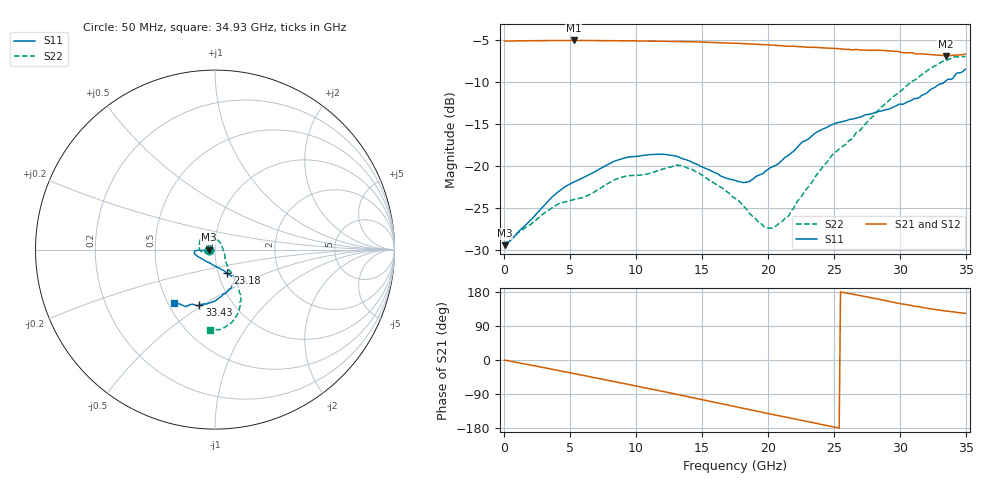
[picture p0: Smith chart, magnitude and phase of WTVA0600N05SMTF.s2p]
! 50 ohm 2-Port S-parameters measured by Modelithics Inc support@modelithics.com  Tampa, FL USA 813-866-6335 (February 2024)
! Smiths Interconnect,  6dB P/N: WTVA0600N05SMTF, Temperature: 50 C
! Board: 10 mil Rogers 4350B, Mounting Pad Dimensions: Length: 15 mils, Width: 25 mils, Gap: 40 mils.
# Hz S RI R 50
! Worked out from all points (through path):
!   352 points, 50 MHz to 34.93 GHz, reference 50 ohm
!   highest |S21| = -5.06 dB at 5.274 GHz (marker M1); lowest = -6.9 dB at 33.43 GHz (marker M2)
!   group delay of S21, straight-line fit = 19.5 ps
!   lowest |S11| = -29.5 dB at 50 MHz (marker M3), VSWR 1.07, Z = 46.7 - j0.0123 ohm
!   |S11| at or under -10 dB: start of sweep to 33.34 GHz
!   |S22| runs from -29.5 to -7.0 dB; largest |S21 - S12| = 0.006
!   S11 on the Smith chart (normalised r, x): 50 MHz: 0.93, -0.00; 23.18 GHz: 1.11, -0.30; 33.43 GHz: 0.70, -0.48; 34.93 GHz: 0.54, -0.37
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5e7  -0.0337 -0.000131  0.5542 -0.00272  0.5539 -0.00284  -0.0333 -0.00208
1.0955e9  -0.0404 -0.00414  0.5509 -0.0696  0.5506 -0.0696  -0.0395 -0.00774
3.4835e9  -0.0633 -0.00499  0.5121 -0.2202  0.5115 -0.2205  -0.0529 -0.0158
5.2745e9  -0.0801 -0.00379  0.4535 -0.3256  0.4532 -0.325  -0.0609 -0.0164
5.8715e9  -0.0842 -0.00353  0.4288 -0.3571  0.4284 -0.3568  -0.0626 -0.0154
8.757e9  -0.1092 -0.00599  0.2792 -0.4805  0.2783 -0.4804  -0.0849 -0.00182
1.1742e10  -0.1158 -0.0196  0.087 -0.5452  0.0859 -0.5448  -0.0864 0.0382
1.36325e10  -0.1057 -0.0303  -0.0444 -0.5486  -0.0452 -0.548  -0.0726 0.0679
1.48265e10  -0.0916 -0.0405  -0.1267 -0.5321  -0.1276 -0.5312  -0.0513 0.074
1.7513e10  -0.0485 -0.0661  -0.293 -0.4513  -0.293 -0.4506  -0.00151 0.064
1.8508e10  -0.0244 -0.0767  -0.3448 -0.406  -0.3449 -0.4053  0.0181 0.05
1.9702e10  0.00103 -0.0914  -0.3981 -0.3455  -0.3979 -0.3448  0.0361 0.0242
2.0299e10  0.0113 -0.0979  -0.4213 -0.3118  -0.4209 -0.3115  0.0408 0.0122
2.1493e10  0.0348 -0.1097  -0.4547 -0.2439  -0.4546 -0.2429  0.0483 -0.0128
2.31845e10  0.0687 -0.131  -0.4884 -0.1421  -0.4878 -0.1422  0.0568 -0.0529
2.33835e10  0.0734 -0.134  -0.492 -0.1301  -0.4915 -0.13  0.0578 -0.0577
2.4876e10  0.094 -0.1495  -0.5 -0.0362  -0.4995 -0.0353  0.0696 -0.0939
2.63685e10  0.1044 -0.1588  -0.4881 0.051  -0.4874 0.0519  0.0827 -0.1196
2.91545e10  0.0973 -0.1954  -0.4379 0.2061  -0.4354 0.2098  0.1297 -0.2091
3.19405e10  0.023 -0.2688  -0.3388 0.3146  -0.3375 0.3152  0.1344 -0.3386
3.3433e10  -0.087 -0.3085  -0.2854 0.3505  -0.2828 0.3519  0.0735 -0.4171
3.49255e10  -0.2292 -0.2984  -0.2541 0.3867  -0.2536 0.3861  -0.0284 -0.4474
